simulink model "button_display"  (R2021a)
settings: Solver=FixedStepDiscrete  StartTime=0.0  StopTime=Inf  RelTol=1e-3  EnableMultiTasking=on
libraries: c2806xlib x10, simulink x1

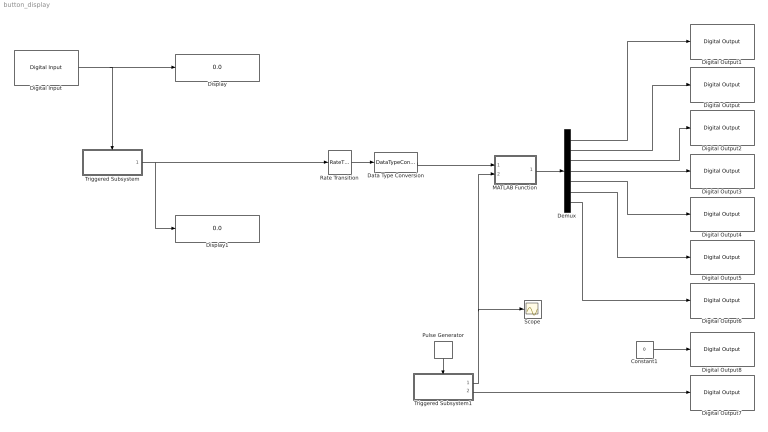
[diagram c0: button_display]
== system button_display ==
  Constant1 : Constant  Value=0
  Data Type Conversion : DataTypeConversion  OutDataTypeStr=uint16
  Demux : Demux  Outputs=7
  Digital Input : c2806xlib/Digital Input  GPIO_Number=GPIO50~GPIO55  GPIO_Bit0=off  GPIO_Bit1=off  GPIO_Bit2=off  GPIO_Bit3=off  GPIO_Bit4=on  GPIO_Bit5=off  GPIO_Bit6=off  GPIO_Bit7=off  sampleTime=0.1  dataType=auto  GPIO_Bit0_Qualification=Sync to SYSCLKOUT  GPIO_Bit1_Qualification=Sync to SYSCLKOUT  GPIO_Bit2_Qualification=Sync to SYSCLKOUT  GPIO_Bit3_Qualification=Sync to SYSCLKOUT  GPIO_Bit4_Qualification=Sync to SYSCLKOUT  GPIO_Bit5_Qualification=Sync to SYSCLKOUT  GPIO_Bit6_Qualification=Sync to SYSCLKOUT  GPIO_Bit7_Qualification=Sync to SYSCLKOUT  Qualification_Period=-1
  Digital Output : c2806xlib/Digital Output  GPIO_Number=GPIO16~GPIO23  GPIO_Bit0=off  GPIO_BIT0_Toggle=off  GPIO_Bit1=off  GPIO_BIT1_Toggle=off  GPIO_Bit2=off  GPIO_BIT2_Toggle=off  GPIO_Bit3=on  GPIO_BIT3_Toggle=off  GPIO_Bit4=off  GPIO_BIT4_Toggle=off  GPIO_Bit5=off  GPIO_BIT5_Toggle=off  GPIO_Bit6=off  GPIO_BIT6_Toggle=off  GPIO_Bit7=off  GPIO_BIT7_Toggle=off
  Digital Output1 : c2806xlib/Digital Output  GPIO_Number=GPIO50~GPIO55  GPIO_Bit0=off  GPIO_BIT0_Toggle=off  GPIO_Bit1=off  GPIO_BIT1_Toggle=off  GPIO_Bit2=on  GPIO_BIT2_Toggle=off  GPIO_Bit3=off  GPIO_BIT3_Toggle=off  GPIO_Bit4=off  GPIO_BIT4_Toggle=off  GPIO_Bit5=off  GPIO_BIT5_Toggle=off  GPIO_Bit6=off  GPIO_BIT6_Toggle=off  GPIO_Bit7=off  GPIO_BIT7_Toggle=off
  Digital Output2 : c2806xlib/Digital Output  GPIO_Number=GPIO8~GPIO15  GPIO_Bit0=off  GPIO_BIT0_Toggle=off  GPIO_Bit1=off  GPIO_BIT1_Toggle=off  GPIO_Bit2=off  GPIO_BIT2_Toggle=off  GPIO_Bit3=off  GPIO_BIT3_Toggle=off  GPIO_Bit4=off  GPIO_BIT4_Toggle=off  GPIO_Bit5=on  GPIO_BIT5_Toggle=off  GPIO_Bit6=off  GPIO_BIT6_Toggle=off  GPIO_Bit7=off  GPIO_BIT7_Toggle=off
  Digital Output3 : c2806xlib/Digital Output  GPIO_Number=GPIO0~GPIO7  GPIO_Bit0=off  GPIO_BIT0_Toggle=off  GPIO_Bit1=off  GPIO_BIT1_Toggle=off  GPIO_Bit2=off  GPIO_BIT2_Toggle=off  GPIO_Bit3=off  GPIO_BIT3_Toggle=off  GPIO_Bit4=off  GPIO_BIT4_Toggle=off  GPIO_Bit5=on  GPIO_BIT5_Toggle=off  GPIO_Bit6=off  GPIO_BIT6_Toggle=off  GPIO_Bit7=off  GPIO_BIT7_Toggle=off
  Digital Output4 : c2806xlib/Digital Output  GPIO_Number=GPIO16~GPIO23  GPIO_Bit0=off  GPIO_BIT0_Toggle=off  GPIO_Bit1=on  GPIO_BIT1_Toggle=off  GPIO_Bit2=off  GPIO_BIT2_Toggle=off  GPIO_Bit3=off  GPIO_BIT3_Toggle=off  GPIO_Bit4=off  GPIO_BIT4_Toggle=off  GPIO_Bit5=off  GPIO_BIT5_Toggle=off  GPIO_Bit6=off  GPIO_BIT6_Toggle=off  GPIO_Bit7=off  GPIO_BIT7_Toggle=off
  Digital Output5 : c2806xlib/Digital Output  GPIO_Number=GPIO0~GPIO7  GPIO_Bit0=off  GPIO_BIT0_Toggle=off  GPIO_Bit1=off  GPIO_BIT1_Toggle=off  GPIO_Bit2=off  GPIO_BIT2_Toggle=off  GPIO_Bit3=off  GPIO_BIT3_Toggle=off  GPIO_Bit4=on  GPIO_BIT4_Toggle=off  GPIO_Bit5=off  GPIO_BIT5_Toggle=off  GPIO_Bit6=off  GPIO_BIT6_Toggle=off  GPIO_Bit7=off  GPIO_BIT7_Toggle=off
  Digital Output6 : c2806xlib/Digital Output  GPIO_Number=GPIO40~GPIO44  GPIO_Bit0=off  GPIO_BIT0_Toggle=off  GPIO_Bit1=off  GPIO_BIT1_Toggle=off  GPIO_Bit2=off  GPIO_BIT2_Toggle=off  GPIO_Bit3=off  GPIO_BIT3_Toggle=off  GPIO_Bit4=on  GPIO_BIT4_Toggle=off  GPIO_Bit5=off  GPIO_BIT5_Toggle=off  GPIO_Bit6=off  GPIO_BIT6_Toggle=off  GPIO_Bit7=off  GPIO_BIT7_Toggle=off
  Digital Output7 : c2806xlib/Digital Output  GPIO_Number=GPIO0~GPIO7  GPIO_Bit0=on  GPIO_BIT0_Toggle=off  GPIO_Bit1=on  GPIO_BIT1_Toggle=off  GPIO_Bit2=on  GPIO_BIT2_Toggle=off  GPIO_Bit3=on  GPIO_BIT3_Toggle=off  GPIO_Bit4=off  GPIO_BIT4_Toggle=off  GPIO_Bit5=off  GPIO_BIT5_Toggle=off  GPIO_Bit6=off  GPIO_BIT6_Toggle=off  GPIO_Bit7=off  GPIO_BIT7_Toggle=off
  Digital Output8 : c2806xlib/Digital Output  GPIO_Number=GPIO16~GPIO23  GPIO_Bit0=on  GPIO_BIT0_Toggle=off  GPIO_Bit1=off  GPIO_BIT1_Toggle=off  GPIO_Bit2=off  GPIO_BIT2_Toggle=off  GPIO_Bit3=off  GPIO_BIT3_Toggle=off  GPIO_Bit4=off  GPIO_BIT4_Toggle=off  GPIO_Bit5=off  GPIO_BIT5_Toggle=off  GPIO_Bit6=off  GPIO_BIT6_Toggle=off  GPIO_Bit7=off  GPIO_BIT7_Toggle=off
  Display : Display
  Display1 : Display
  MATLAB Function : MATLAB Function  TreatAsAtomicUnit=on
  Pulse Generator : DiscretePulseGenerator  SampleTime=0.0005
  Rate Transition : RateTransition
  Scope : Scope
  Triggered Subsystem : Subsystem  TreatAsAtomicUnit=on
  Triggered Subsystem1 : Subsystem  TreatAsAtomicUnit=on
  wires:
  Digital Input/1 -> Triggered Subsystem/Trigger, Display/1
  Triggered Subsystem/1(u) -> Display1/1, Rate Transition/1
  Demux/1 -> Digital Output1/1
  Demux/2 -> Digital Output/1
  Demux/3 -> Digital Output2/1
  Demux/4 -> Digital Output3/1
  Demux/5 -> Digital Output4/1
  Demux/6 -> Digital Output5/1
  Demux/7 -> Digital Output6/1
  MATLAB Function/1(y) -> Demux/1
  Constant1/1 -> Digital Output8/1
  Pulse Generator/1 -> Triggered Subsystem1/Trigger
  Triggered Subsystem1/2(digit) -> Digital Output7/1
  Triggered Subsystem1/1(n) -> Scope/1, MATLAB Function/2(digit)
  Rate Transition/1 -> Data Type Conversion/1
  Data Type Conversion/1 -> MATLAB Function/1(num)

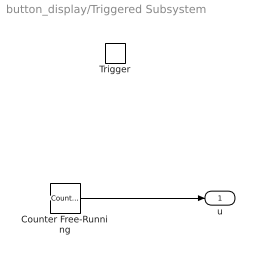
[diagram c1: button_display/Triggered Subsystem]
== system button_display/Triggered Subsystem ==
  Trigger : TriggerPort  VariantControl=(inherit)
  Counter Free-Running : simulink/Sources/Counter Free-Running  NumBits=12  tsamp=-1
  u : Outport
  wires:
  Counter Free-Running/1 -> u/1

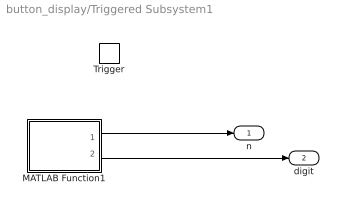
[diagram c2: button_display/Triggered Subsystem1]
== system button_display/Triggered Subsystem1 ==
  Trigger : TriggerPort  VariantControl=(inherit)
  MATLAB Function1 : MATLAB Function  TreatAsAtomicUnit=on
  n : Outport
  digit : Outport  Port=2
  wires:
  MATLAB Function1/1(nn) -> n/1
  MATLAB Function1/2(digit) -> digit/1

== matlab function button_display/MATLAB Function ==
function y = fcn(num,digit)

  segments = [0 0 0 0 0 0 0]
  x = uint16(0)
  

    
    k   = idivide(num,1000);
    num = num - k*1000;
        
    h  = idivide( num,100 );
    num = num - h*100;
        
    da = idivide( num,10 );
    num = num - da*10;
      
    u  = num;
        
        
    switch digit 
        case 0
            % u
            x = u;
        case 1
            % da
            x = da;
        case 2
            % h
            x = h;
        case 3
            % k
            x = k;
            
    end
        
    
switch x
    case 0
        segments = [1 1 1 1 1 1 0]
    case 1
        segments = [0 1 1 0 0 0 0]
    case 2
        segments = [1 1 0 1 1 0 1]
    case 3
        segments = [1 1 1 1 0 0 1]
    case 4
        segments = [0 1 1 0 0 1 1]
    case 5
        segments = [1 0 1 1 0 1 1]
    case 6
        segments = [1 0 1 1 1 1 1]
    case 7
        segments = [1 1 1 0 0 0 0]
    case 8
        segments = [1 1 1 1 1 1 1]
    case 9
        segments = [1 1 1 0 0 1 1]
    otherwise
        segments = [0 0 0 0 0 0 1]

end


y = segments;

== matlab function button_display/Triggered
Subsystem1/MATLAB Function1 ==
function [nn, digit]= fcn
    persistent n
    digit = [1 0 0 0]     
    if isempty(n)
        n = 0;
    else
        n = n+1;
    end
    
    if n>3
        n=0;
    end
  
    switch n
        case 3
            digit = [0 0 0 1]
        case 2
            digit = [0 0 1 0]
        case 1
            digit = [0 1 0 0]
        case 0
            digit = [1 0 0 0]
    end
    nn=n
y = [nn,digit];
